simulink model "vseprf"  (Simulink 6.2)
settings: Solver=ode45  StartTime=0.0  StopTime=5  RelTol=1e-3  AbsTol=1e-3

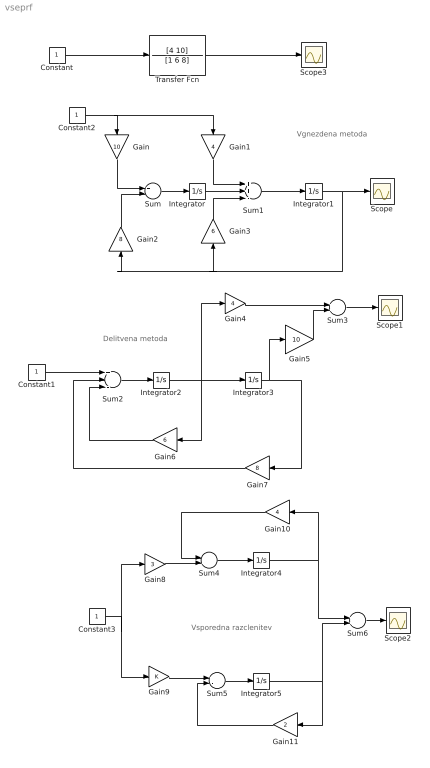
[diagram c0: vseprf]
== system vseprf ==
  note: Vgnezdena metoda
  note: Delitvena metoda
  note: Vsporedna razclenitev
  Constant{,1..3} (4 alike) : Constant
  Gain : Gain  Orientation=down  Gain=10
  Gain1 : Gain  Orientation=down  Gain=4
  Gain10 : Gain  Orientation=left  Gain=4
  Gain11 : Gain  Orientation=left  Gain=2
  Gain2 : Gain  Orientation=up  Gain=8
  Gain3 : Gain  Orientation=up  Gain=6
  Gain4 : Gain  Gain=4
  Gain5 : Gain  Gain=10
  Gain6 : Gain  Orientation=left  Gain=6
  Gain7 : Gain  Orientation=left  Gain=8
  Gain8 : Gain  Gain=3
  Gain9 : Gain
  Integrator{,1..5} (6 alike) : Integrator
  Scope{,1..3} (4 alike) : Scope
  Sum : Sum  Inputs=+-
  Sum1 : Sum  Inputs=++-
  Sum2 : Sum  Inputs=+--
  Sum3 : Sum
  Sum4 : Sum  Inputs=-+
  Sum5 : Sum  Inputs=+-
  Sum6 : Sum
  Transfer Fcn : TransferFcn  Numerator=[4 10]  Denominator=[1 6 8]
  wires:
  Gain9/1 -> Sum5/1
  Sum5/1 -> Integrator5/1
  Integrator5/1 -> Sum6/2, Gain11/1
  Gain11/1 -> Sum5/2
  Constant/1 -> Transfer Fcn/1
  Transfer Fcn/1 -> Scope3/1
  Gain/1 -> Sum/1
  Sum/1 -> Integrator/1
  Sum1/1 -> Integrator1/1
  Gain2/1 -> Sum/2
  Gain3/1 -> Sum1/3
  Integrator/1 -> Sum1/2
  Gain1/1 -> Sum1/1
  Integrator1/1 -> Gain3/1, Gain2/1, Scope/1
  Sum2/1 -> Integrator2/1
  Integrator2/1 -> Integrator3/1, Gain6/1, Gain4/1
  Gain6/1 -> Sum2/3
  Gain7/1 -> Sum2/2
  Gain4/1 -> Sum3/1
  Integrator3/1 -> Gain7/1, Gain5/1
  Gain5/1 -> Sum3/2
  Sum3/1 -> Scope1/1
  Gain8/1 -> Sum4/2
  Sum4/1 -> Integrator4/1
  Integrator4/1 -> Sum6/1, Gain10/1
  Gain10/1 -> Sum4/1
  Sum6/1 -> Scope2/1
  Constant1/1 -> Sum2/1
  Constant2/1 -> Gain1/1, Gain/1
  Constant3/1 -> Gain8/1, Gain9/1
